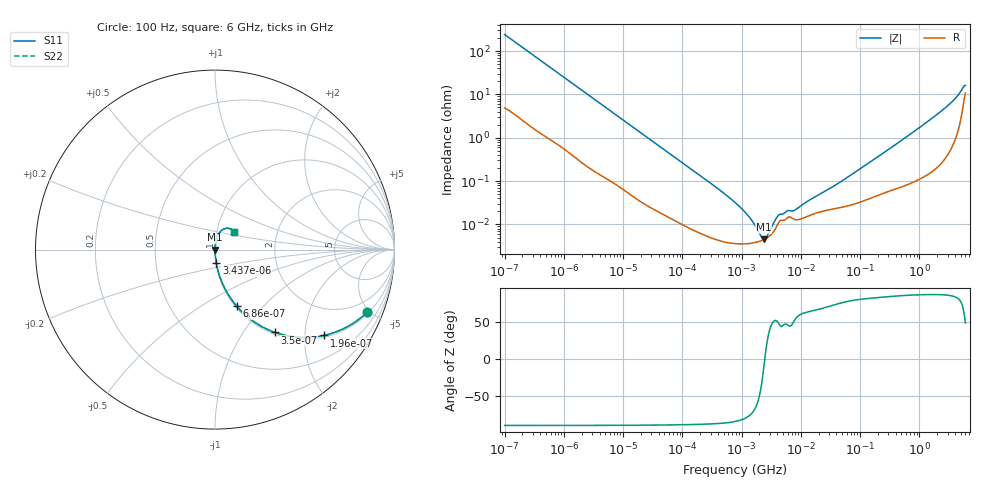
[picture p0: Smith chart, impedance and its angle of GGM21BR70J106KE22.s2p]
!Murata Part Number: GGM21BR70J106KE22
!These Parameters are Measured in Series Mode Connection
!Data Generated on Jun 19, 2026
!  o--ll--o
!Port1  Port2
!  o------o
!Operation Temp=25[degC], DC Bias Voltage=0[V]
!Freq. Start=100[Hz] Stop=6[GHz] 401[Steps]
# Hz S RI R 50
!Freq.(Hz) S11(Real) S11(Imag) S21(Real) S21(Imag) S12(Real) S12(Imag) S22(Real) S22(Imag)
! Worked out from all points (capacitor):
!   401 points, 100 Hz to 6 GHz, reference 50 ohm
!   read as one part in series: C = 6.55 uF near 109 Hz
!   lowest |Z| = 4.57 mohm at 2.373 MHz (marker M1)
!   series resonance near 2.462 MHz, so ESL is about 640 pH
!   S11 on the Smith chart (normalised r, x): 100 Hz: 1.10, -4.83; 196 Hz: 1.05, -2.49; 350 Hz: 1.03, -1.40; 686 Hz: 1.02, -0.72; 3.437 kHz: 1.00, -0.15; 6 GHz: 1.21, +0.24
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100  0.8487 -0.3483  0.1513 0.3483  0.1513 0.3483  0.8487 -0.3483
196  0.6067 -0.4782  0.3933 0.4782  0.3933 0.4782  0.6067 -0.4782
350  0.3334 -0.4613  0.6666 0.4613  0.6666 0.4613  0.3334 -0.4613
686  0.1212 -0.3155  0.8788 0.3155  0.8788 0.3155  0.1212 -0.3155
2008  0.018 -0.1229  0.982 0.1229  0.982 0.1229  0.018 -0.1229
3437  0.007 -0.0731  0.993 0.0731  0.993 0.0731  0.007 -0.0731
40335  0.000235 -0.00652  0.9998 0.00652  0.9998 0.00652  0.000235 -0.00652
316350  4.9e-05 -0.000849  1 0.000849  1 0.000849  4.9e-05 -0.000849
774597  3.63e-05 -0.000321  1 0.000321  1 0.000321  3.63e-05 -0.000321
1108252  3.58e-05 -0.000199  1 0.000199  1 0.000199  3.58e-05 -0.000199
1658239  3.82e-05 -9.17e-05  1 9.17e-05  1 9.17e-05  3.82e-05 -9.17e-05
2372521  4.49e-05 -8.5e-06  1 8.5e-06  1 8.5e-06  4.49e-05 -8.5e-06
3245845  6.11e-05 6.61e-05  0.9999 -6.61e-05  0.9999 -6.61e-05  6.11e-05 6.61e-05
4440638  0.000121 0.000122  0.9999 -0.000122  0.9999 -0.000122  0.000121 0.000122
6075234  0.000147 0.000148  0.9999 -0.000148  0.9999 -0.000148  0.000147 0.000148
7947587  0.00013 0.000172  0.9999 -0.000172  0.9999 -0.000172  0.00013 0.000172
1.555665e7  0.00017 0.000359  0.9998 -0.000359  0.9998 -0.000359  0.00017 0.000359
4.764863e7  0.000248 0.000945  0.9998 -0.000945  0.9998 -0.000945  0.000248 0.000945
3.124326e8  0.000616 0.00551  0.9994 -0.00551  0.9994 -0.00551  0.000616 0.00551
2.450438e9  0.00458 0.0428  0.9954 -0.0428  0.9954 -0.0428  0.00458 0.0428
4.385646e9  0.0204 0.0879  0.9796 -0.0879  0.9796 -0.0879  0.0204 0.0879
6e9  0.1075 0.0972  0.8925 -0.0972  0.8925 -0.0972  0.1075 0.0972
